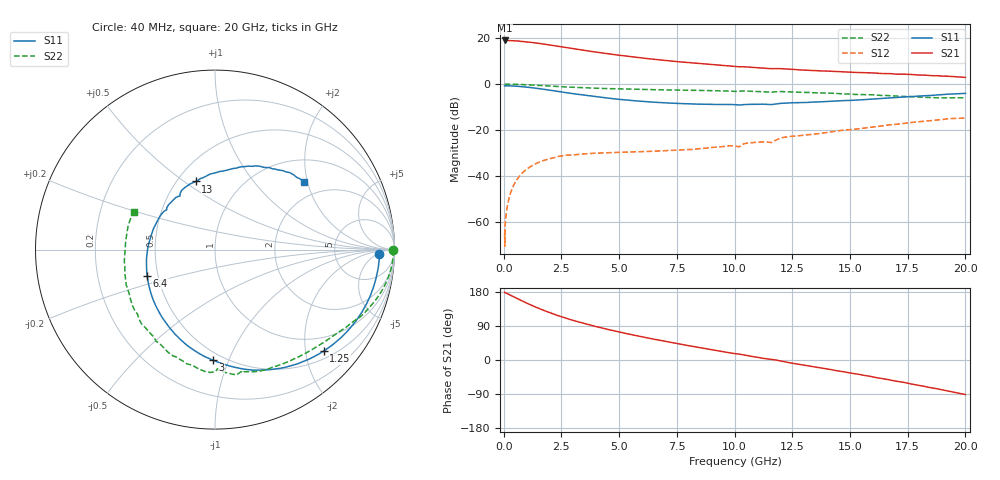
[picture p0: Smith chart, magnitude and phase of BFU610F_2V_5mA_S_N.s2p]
! Filename:  P:\Prog\Test\Noise\ATS_data\Testdata_Net\SplitFiles\BFU610_2W_A5_HighFreq_2V_5mA_D.s2p
! Date/Time: Wed 10/Aug/2011 16:55:59
! BFU610_2W_A5_HighFreq_2V_1mA_10mA_Bias4_R.s2p
! MDIF S-parameter v. bias file
! BFU610_2W_A5_HighFreq_2V_1mA_10mA
! Date/time Mon Aug 08 14:20:39 2011
! VAR V_out= 2.0002
! VAR I_out= 4.9950
! VAR V_in= 0.9009
! VAR I_in= 0.0406
! Device data file deembeded for feedlines and parallel
! Original file: \SplitFiles\BFU610_2W_A5_HighFreq_2V_5mA_R.s2p
! Feed-files: PR003V01_101208_Feed1.s2p, PR003V01_101208_Feed2.s2p
! Parallel-file: PR003V01_101208_Par.s2p
# MHz S MA R 50
!  Freq-MHz  S11-mag  S11-arg  S21-mag  S21-arg  S12-mag  S12-arg  S22-mag  S22-arg
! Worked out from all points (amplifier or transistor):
!   167 points, 40 MHz to 20 GHz, reference 50 ohm
!   highest |S21| = 19.0 dB at 40 MHz (marker M1)
!   |S21| within 3 dB of that: start of sweep to 2.629 GHz
!   unconditionally stable (mu >= 1): 4.616 GHz to 18.14 GHz
!   at 550 MHz: K = 0.07, MSG = 30.5 dB, |S12| = -42.1 dB
!   at 4.2 GHz: K = 0.90, MSG = 21.9 dB, |S12| = -30.1 dB
!   at 20 GHz: K = 0.88, MSG = 8.8 dB, |S12| = -14.8 dB
!   lowest NFmin = 1.25 dB at 400 MHz
!   S11 on the Smith chart (normalised r, x): 40 MHz: 21, -6; 1.25 GHz: 0.66, -2.38; 3 GHz: 0.44, -0.88; 6.4 GHz: 0.44, -0.15; 13 GHz: 0.62, +0.55; 20 GHz: 1.54, +1.91
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40  0.9165 -1.4  8.923 178.5  0.000555 84.2  0.9908 -0.2
50  0.9092 -2.0  8.889 178.6  0.0002903 100.6  0.9913 -0.5
60  0.9161 -1.9  8.912 177.7  0.0007742 105.0  0.9922 -0.6
120  0.9156 -4.3  8.887 176.1  0.001613 89.7  0.9926 -1.4
360  0.9081 -12.9  8.811 168.8  0.005122 85.6  0.9899 -4.6
800  0.8761 -28.3  8.515 155.7  0.01135 75.3  0.9739 -10.2
1250  0.8284 -43.1  8.029 143.2  0.01683 66.0  0.9495 -15.3
1650  0.7797 -55.4  7.553 133.0  0.0208 58.9  0.9256 -19.4
2000  0.7352 -65.5  7.114 124.8  0.02355 53.5  0.9056 -22.8
2500  0.6718 -78.9  6.471 114.1  0.02693 47.1  0.8723 -27.1
3000  0.6167 -91.0  5.896 104.6  0.0285 41.1  0.8485 -30.7
3400  0.5791 -100.2  5.491 97.9  0.02964 38.8  0.8302 -33.5
4000  0.5282 -113.2  4.966 88.2  0.03104 35.5  0.8088 -37.5
4700  0.481 -127.3  4.442 78.1  0.032 33.2  0.7892 -42.1
6400  0.4051 -159.0  3.509 56.2  0.03405 32.4  0.7545 -53.2
6800  0.3931 -166.1  3.344 51.5  0.03464 32.9  0.7485 -55.7
8600  0.3627 164.4  2.772 31.5  0.03925 37.4  0.7243 -67.8
10200  0.3484 140.6  2.378 15.6  0.04258 42.0  0.6944 -77.6
13000  0.3947 105.9  2.021 -13.4  0.07642 36.9  0.6557 -102.0
13400  0.4042 101.6  1.966 -17.4  0.08022 35.6  0.6462 -106.0
16800  0.5022 67.9  1.681 -53.5  0.1295 16.2  0.5548 -146.2
20000  0.6247 37.3  1.395 -91.2  0.1819 -15.2  0.5003 154.9
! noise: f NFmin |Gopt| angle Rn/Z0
400  1.253  0.546  3.19  0.4886
800  1.285  0.5311  7.445  0.4876
1250  1.323  0.5153  12.17  0.4847
1700  1.364  0.5001  16.82  0.4799
2150  1.407  0.4853  21.39  0.4734
2700  1.464  0.4671  26.88  0.4634
3600  1.565  0.4363  35.67  0.4431
4500  1.677  0.4023  44.33  0.4188
5800  1.856  0.3443  57.19  0.3797
8000  2.208  0.2174  86.43  0.3131
